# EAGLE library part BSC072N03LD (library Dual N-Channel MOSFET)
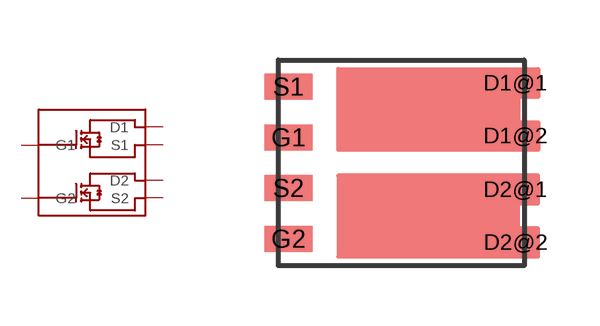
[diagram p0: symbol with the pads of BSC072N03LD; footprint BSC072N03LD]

Designator prefix Q

## BSC072N03LD  [BSC072N03LD]
D1@1  D1
D1@2  D1
D2@1  D2
D2@2  D2
G1  G1
G2  G2
S1  S1
S2  S2

## Footprint BSC072N03LD (pad centres in mm)
smd 1.2 x 0.65: D1@1 2.857,2.009; D1@2 2.857,0.689; D2@1 2.857,-0.657; D2@2 2.864,-1.98; G1 -2.825,0.634; G2 -2.825,-1.905; S1 -2.825,1.905; S2 -2.825,-0.634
